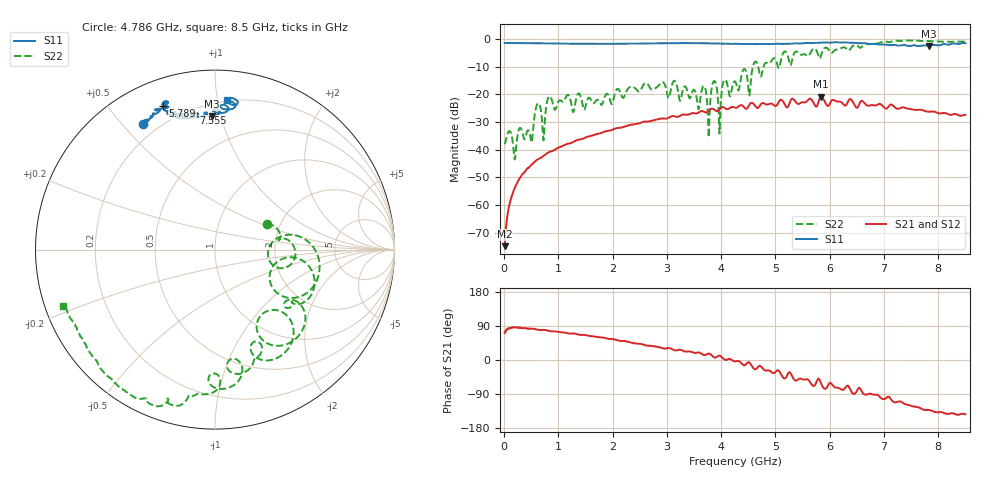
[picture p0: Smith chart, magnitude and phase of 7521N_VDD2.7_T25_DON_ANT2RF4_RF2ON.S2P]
!Agilent Technologies,E5071C,MY46417908,A.11.23
!Date: Thu Jul 30 15:13:46 2020
!Data & Calibration Information:
!Freq	S11:SOLT2(ON)	S21:SOLT2(ON)	S12:SOLT2(ON)	S22:SOLT2(ON)
!PortZ  Port1:50+j0  Port2:50+j0
!Above PortZ is port z conversion or system Z0 setting when saving the data.
!When reading, reference impedance value at option line is always used.
# Hz S dB R 50
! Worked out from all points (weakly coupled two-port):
!   1601 points, 10 MHz to 8.5 GHz, reference 50 ohm
!   highest |S21| = -20.87 dB at 5.842 GHz (marker M1); lowest = -74.9 dB at 10 MHz (marker M2)
!   lowest |S11| = -2.6 dB at 7.821 GHz (marker M3), VSWR 6.79, Z = 14.1 + j46.7 ohm
!   |S11| at or under -10 dB: nowhere
!   |S22| runs from -43.6 to -0.6 dB; largest |S21 - S12| = 0.0024
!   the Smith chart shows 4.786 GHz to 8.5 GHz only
!   S11 on the Smith chart (normalised r, x): 4.786 GHz: 0.14, +0.57; 5.789 GHz: 0.12, +0.70; 7.555 GHz: 0.22, +0.83; 8.5 GHz: 0.19, +1.07
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1e7  -1.45 179.9  -74.89 72.2  -74.91 66.2  -38.01 -3.7
3.496e8  -1.53 174.8  -48.65 84.1  -48.69 83.7  -34.74 -87.4
5.034812e8  -1.55 172.6  -45.51 82.5  -45.52 82.5  -37.42 -66.6
6.25525e8  -1.58 170.7  -43.49 79.7  -43.49 80.0  -23.23 -79.2
7.3165e8  -1.60 169.5  -42.21 79.6  -42.26 79.8  -35.92 -65.3
8.324688e8  -1.62 167.7  -40.90 76.6  -40.87 76.6  -20.75 -86.9
1.426769e9  -1.76 158.8  -36.22 66.0  -36.22 65.9  -21.87 -145.6
2.843538e9  -1.56 140.2  -28.97 34.1  -28.99 34.1  -16.95 169.7
3.681925e9  -1.59 130.8  -26.27 13.1  -26.27 12.9  -16.95 103.1
3.766825e9  -1.58 131.2  -26.16 16.9  -26.17 16.8  -34.52 80.4
3.862338e9  -1.66 129.3  -25.39 7.5  -25.40 7.4  -15.34 106.6
3.968462e9  -1.68 129.1  -25.47 11.5  -25.48 11.3  -34.17 83.3
4.058669e9  -1.73 127.6  -24.84 1.4  -24.86 1.3  -14.81 92.0
4.255e9  -1.72 125.5  -24.84 -3.8  -24.86 -4.0  -15.38 55.9
4.785625e9  -1.84 119.9  -23.24 -25.2  -23.22 -25.6  -9.79 26.5
5.671769e9  -1.52 111.3  -22.07 -65.6  -22.04 -65.9  -4.05 -36.6
5.788506e9  -1.40 109.8  -23.11 -49.2  -23.04 -49.3  -5.94 -62.5
5.841569e9  -1.35 109.6  -20.87 -62.0  -20.82 -62.2  -5.86 -42.9
7.088538e9  -2.20 106.6  -24.34 -97.1  -24.16 -95.6  -1.20 -107.7
7.555488e9  -2.27 98.7  -25.61 -123.1  -25.51 -121.0  -0.61 -123.9
7.8208e9  -2.58 91.5  -26.33 -131.9  -26.40 -130.1  -0.78 -134.8
8.5e9  -1.54 85.4  -27.40 -143.4  -27.47 -143.6  -0.89 -159.7
